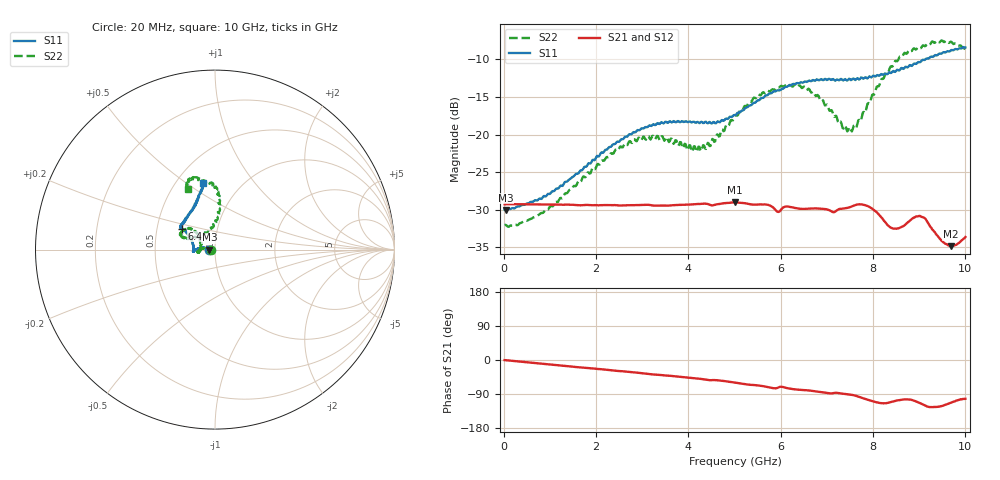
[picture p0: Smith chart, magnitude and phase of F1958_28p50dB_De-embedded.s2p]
! Integrated Device Technology
! Corporate Headquarters
! 6024 Silver Creek Valley Road
! San Jose, CA 95138  USA
! Phone:  1-408-284-8200
! Toll Free:  1-800-223-1366
! Webpage:  http://www.idt.com/
! Timing and RF Division
! 515 Groton Road, Suite 102
! Westford, MA 01886-6024
! Device:  F1958
! Description: 7-bit 0.25 dB Digital Step Attenuator
! Frequency:  0.001 -  6.000 GHz
! Package:  4x4 mm Thin QFN Plastic Package: 24 pin
! Ports:  2 RF, 12 DC
!  Pin  1  = D0
!  Pin  2  = VDD
!  Pin  3  = VMODE
!  Pin  4  = GND
!  Pin  5  = RF1  =  Port 1
!  Pin  6  = GND
!  Pin  7  = GND
!  Pin  8  = GND
!  Pin  9  = GND
!  Pin 10  = GND
!  Pin 11  = GND
!  Pin 12  = GND
!  Pin 13  = GND
!  Pin 14  = RF2  =  Port 2
!  Pin 15  = GND
!  Pin 16  = LE
!  Pin 17  = CLK
!  Pin 18  = DATA
!  Pin 19  = D6
!  Pin 20  = D5
!  Pin 21  = D4
!  Pin 22  = D3
!  Pin 23  = D2
!  Pin 24  = D1
! State:  114
! Atten State:  28.50 dB
! Voltage:  +3.30 Volts
! Current:  0.258 mA
! Data:  The device was measured on a F1958 evaluation board which has
!  individual transmission lines to the RF pins.  Data was collected
!  using a calibrated network analyzer.  The evaluation board was
!  de-embedded using Automatic Fixture Removal (AFR).
!  The reference plane is the edge of the package pin.
! Misc:
!  Action Tracker AT0419
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# GHz S dB R 50
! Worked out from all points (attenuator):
!   500 points, 20 MHz to 10 GHz, reference 50 ohm
!   highest |S21| = -29.03 dB at 5 GHz (marker M1); lowest = -34.8 dB at 9.68 GHz (marker M2)
!   lowest |S11| = -30.0 dB at 40 MHz (marker M3), VSWR 1.07, Z = 46.9 - j0.0474 ohm
!   |S11| at or under -10 dB: start of sweep to 9.134 GHz
!   |S22| runs from -32.3 to -7.5 dB; largest |S21 - S12| = 0.00031
!   S11 on the Smith chart (normalised r, x): 20 MHz: 0.94, -0.00; 6.4 GHz: 0.67, +0.16; 10 GHz: 0.67, +0.59
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0.02  -30.00 -179.0  -29.28 -0.2  -29.28 -0.2  -32.04 -178.9
0.04  -30.03 -179.1  -29.27 -0.4  -29.27 -0.3  -32.01 -178.5
0.84  -28.41 171.0  -29.31 -9.9  -29.29 -9.9  -30.43 172.1
1.7  -24.74 171.0  -29.40 -19.6  -29.40 -19.6  -25.86 171.0
2.6  -20.53 176.8  -29.41 -30.0  -29.39 -30.0  -21.45 179.2
3.36  -18.58 -175.7  -29.44 -39.3  -29.45 -39.4  -20.52 -169.4
4.24  -18.49 -179.1  -29.24 -49.4  -29.24 -49.4  -21.64 168.9
4.5  -18.54 175.0  -29.42 -53.2  -29.43 -53.4  -21.01 151.3
5  -17.40 161.6  -29.03 -59.5  -29.05 -59.5  -17.65 137.2
5.02  -17.40 160.8  -29.04 -59.9  -29.04 -59.8  -17.42 138.2
5.58  -15.15 150.5  -29.30 -68.4  -29.31 -68.3  -14.68 139.9
5.94  -14.11 148.3  -30.29 -73.0  -30.31 -73.0  -13.74 148.7
6.4  -13.17 147.8  -29.86 -78.5  -29.88 -78.4  -13.45 155.9
6.68  -12.81 146.7  -29.83 -81.4  -29.85 -81.3  -14.38 157.9
7.5  -12.63 138.3  -29.66 -91.2  -29.66 -91.0  -19.04 120.3
7.68  -12.59 135.4  -29.28 -96.5  -29.29 -96.5  -18.11 99.9
7.9  -12.39 128.9  -29.56 -105.6  -29.56 -105.5  -15.81 89.6
8.34  -11.76 118.9  -32.17 -112.8  -32.17 -112.8  -11.56 84.2
8.54  -11.40 115.9  -32.48 -106.5  -32.45 -106.3  -10.13 86.5
9.04  -10.27 106.8  -30.92 -114.9  -30.94 -115.0  -8.49 97.6
9.68  -8.83 100.3  -34.85 -113.0  -34.82 -113.3  -7.65 111.0
10  -8.42 99.8  -33.63 -102.5  -33.74 -102.3  -8.61 114.2
